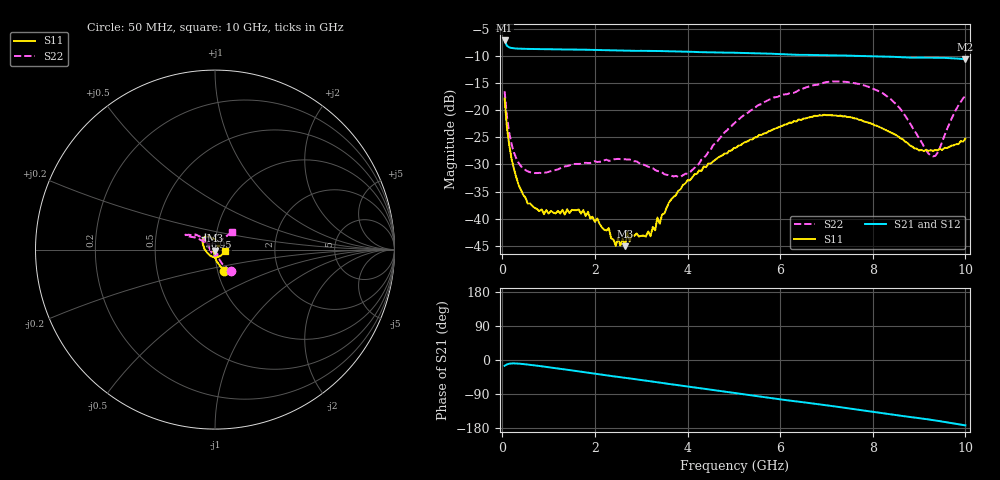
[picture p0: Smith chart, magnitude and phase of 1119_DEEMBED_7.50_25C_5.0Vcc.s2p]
!Hittite Microwave Corp.
!Digital Attenuator/PhaseShifter Rev 1.4.0
!Filename: C:\DATA\DATA\1119_DEEMBED_7.50_25C_5.0Vcc.s2p
!VNA ID: Agilent Technologies,N5224A,MY51441122,A.10.45.03
!Device type:
!2 Port Calibration.
!Temp(C): 25
!Lot Number:
!Serial Number:
!Operator:
!Misc:
!Attenuator:  7.500
# GHZ S DB R 50.0
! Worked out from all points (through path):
!   200 points, 50 MHz to 10 GHz, reference 50 ohm
!   highest |S21| = -7.15 dB at 50 MHz (marker M1); lowest = -10.6 dB at 10 GHz (marker M2)
!   group delay of S21, straight-line fit = 46.5 ps
!   lowest |S11| = -45.1 dB at 2.65 GHz (marker M3), VSWR 1.01, Z = 50.1 - j0.542 ohm
!   |S11| at or under -10 dB: start of sweep to end of sweep
!   |S22| runs from -32.3 to -14.7 dB; largest |S21 - S12| = 0.0013
!   S11 on the Smith chart (normalised r, x): 50 MHz: 1.07, -0.26; 6.95 GHz: 0.88, +0.13; 10 GHz: 1.11, -0.01
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0.05  -17.85 -67.1  -7.15 -15.3  -7.15 -15.3  -16.50 -54.0
0.15  -26.43 -87.2  -8.42 -9.8  -8.42 -9.8  -24.19 -65.9
0.25  -30.76 -95.3  -8.60 -9.0  -8.61 -9.0  -27.77 -64.9
0.55  -37.23 -112.5  -8.71 -12.0  -8.71 -12.0  -31.28 -60.1
0.9  -39.16 -124.0  -8.75 -17.4  -8.75 -17.4  -31.53 -62.9
1.75  -38.39 -127.2  -8.85 -31.7  -8.85 -31.7  -29.72 -78.5
2.3  -41.71 -116.2  -8.95 -41.2  -8.95 -41.3  -29.33 -92.7
2.45  -45.00 -97.1  -9.00 -43.8  -9.01 -43.9  -29.02 -96.6
2.65  -45.06 -75.5  -9.04 -47.0  -9.05 -47.1  -29.05 -103.2
2.7  -42.51 -66.1  -9.05 -47.8  -9.06 -47.9  -29.10 -104.1
2.75  -44.18 -67.6  -9.06 -48.6  -9.06 -48.7  -29.09 -106.5
3.2  -43.24 -13.3  -9.08 -56.1  -9.09 -56.2  -30.60 -124.0
3.35  -39.78 4.0  -9.10 -58.8  -9.11 -58.8  -31.22 -129.4
3.4  -40.92 7.3  -9.10 -59.6  -9.11 -59.6  -31.27 -131.9
3.6  -37.00 22.8  -9.15 -63.2  -9.16 -63.3  -31.98 -141.7
4.05  -32.92 35.7  -9.24 -70.7  -9.25 -70.8  -31.47 179.6
5.05  -26.92 74.6  -9.42 -87.4  -9.44 -87.5  -22.10 136.2
6.7  -21.20 123.8  -9.83 -114.8  -9.85 -114.8  -15.45 150.6
6.95  -20.84 129.2  -9.87 -118.7  -9.89 -118.8  -14.92 152.8
8.35  -23.94 167.4  -10.14 -142.7  -10.15 -142.7  -17.71 148.7
9.3  -27.49 -99.7  -10.31 -158.6  -10.32 -158.6  -28.51 110.3
10  -25.25 -6.5  -10.61 -172.6  -10.62 -172.6  -17.34 46.6
